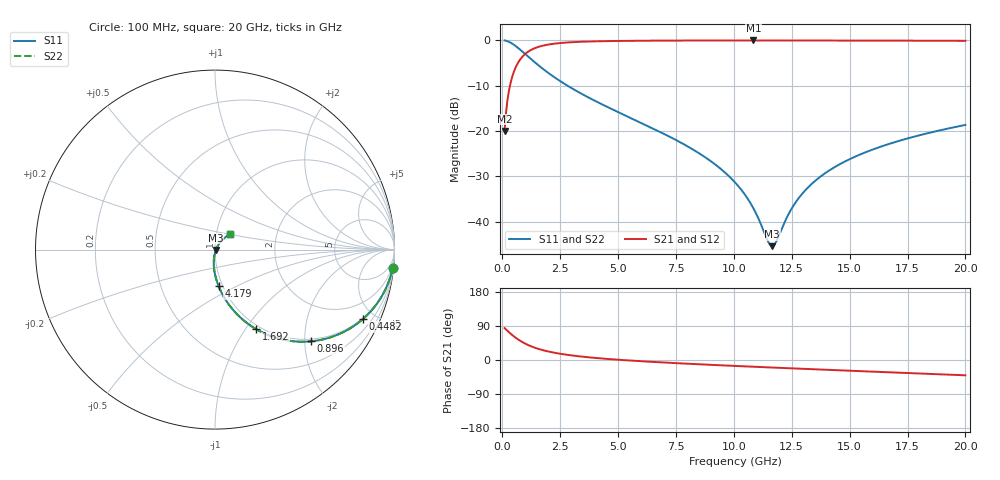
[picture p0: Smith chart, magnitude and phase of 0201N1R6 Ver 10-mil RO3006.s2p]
# GHz S MA R 50
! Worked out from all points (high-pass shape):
!   1601 points, 100 MHz to 20 GHz, reference 50 ohm
!   highest |S21| = -0.05 dB at 10.85 GHz (marker M1); lowest = -20.0 dB at 100 MHz (marker M2)
!   |S21| within 3 dB of the highest: 981.8 MHz to end of sweep
!   lowest |S11| = -45.4 dB at 11.65 GHz (marker M3), VSWR 1.01, Z = 50.5 - j0.191 ohm
!   |S11| at or under -10 dB: 2.813 GHz to end of sweep
!   |S22| runs from -45.4 to 0.0 dB; largest |S21 - S12| = 0
!   S11 on the Smith chart (normalised r, x): 100 MHz: 1, -19; 448.2 MHz: 0.95, -4.30; 896 MHz: 0.95, -2.14; 1.692 GHz: 0.95, -1.12; 4.179 GHz: 0.96, -0.41; 20 GHz: 1.16, +0.20
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0.1  0.995 -5.9  0.1001 84.1  0.1001 84.1  0.995 -5.9
0.2865625  0.9607 -16.6  0.277 73.4  0.277 73.4  0.9607 -16.6
0.44825  0.9111 -25.1  0.4112 64.9  0.4112 64.9  0.9111 -25.1
0.64725  0.8367 -34.2  0.5462 55.7  0.5462 55.7  0.8367 -34.2
0.896  0.7402 -43.7  0.6706 46.2  0.6706 46.2  0.7402 -43.7
1.269125  0.6115 -54.3  0.789 35.5  0.789 35.5  0.6115 -54.3
1.692  0.4982 -62.7  0.8645 27.0  0.8645 27.0  0.4982 -62.7
2.413375  0.3669 -72.2  0.9272 17.4  0.9272 17.4  0.3669 -72.2
3.420812  0.2575 -80.2  0.9627 9.0  0.9627 9.0  0.2575 -80.2
4.1795  0.2043 -84.4  0.9751 4.6  0.9751 4.6  0.2043 -84.4
6.741625  0.09991 -93.3  0.9904 -5.8  0.9904 -5.8  0.09991 -93.3
8.731625  0.05209 -96.7  0.9936 -12.0  0.9936 -12.0  0.05209 -96.7
10.05  0.02722 -94.9  0.9943 -15.7  0.9943 -15.7  0.02722 -94.9
10.846  0.0141 -85.9  0.9944 -17.8  0.9944 -17.8  0.0141 -85.9
11.46787  0.006146 -48.6  0.9943 -19.4  0.9943 -19.4  0.006146 -48.6
11.65444  0.005401 -20.5  0.9943 -19.9  0.9943 -19.9  0.005401 -20.5
11.82856  0.00605 5.8  0.9943 -20.3  0.9943 -20.3  0.00605 5.8
12.58725  0.01525 46.3  0.994 -22.3  0.994 -22.3  0.01525 46.3
13.37081  0.02631 53.2  0.9936 -24.2  0.9936 -24.2  0.02631 53.2
14.73894  0.04541 54.8  0.9927 -27.6  0.9927 -27.6  0.04541 54.8
16.69162  0.07201 52.6  0.9907 -32.4  0.9907 -32.4  0.07201 52.6
20  0.1168 46.2  0.9858 -40.4  0.9858 -40.4  0.1168 46.2
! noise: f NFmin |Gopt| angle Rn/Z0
0.1  0.000971  0.9574  0.7399  0.005137
2.301  0.005359  0.8261  4.398  0.006468
4.515  0.008286  0.7844  8.083  0.007856
6.729  0.01081  0.7578  11.77  0.008936
8.943  0.01311  0.7383  15.44  0.009851
11.14  0.01527  0.7233  19.06  0.01066
13.36  0.01735  0.7113  22.67  0.0114
15.57  0.01937  0.7016  26.23  0.01208
17.79  0.02134  0.6938  29.75  0.01273
20  0.0233  0.6875  33.23  0.01334
